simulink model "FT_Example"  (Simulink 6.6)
settings: Solver=FixedStepDiscrete  StartTime=0.0  StopTime=10  FixedStep=Ts  RelTol=1e-3
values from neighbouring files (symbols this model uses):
  Ts = 1/30    (= 0.0333333333333)    [setup.m]
libraries: RobotLibrary x2

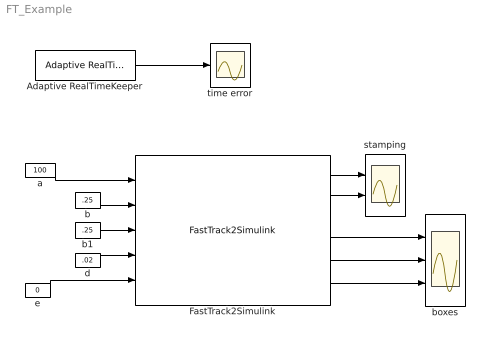
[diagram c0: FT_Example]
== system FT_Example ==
  Adaptive RealTimeKeeper : RobotLibrary/Adaptive RealTimeKeeper  Tag=AdaptiveRealTimeKeeper  Description=|  Priority=0  SystemSampleTime=-1  Ts=Ts
      | This block attempts to synchronize the simulation clock with real time.                                                                                                            
      |                                                                                                                                                                                    
      | The output provides the time-keeping err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
  FastTrack2Simulink : RobotLibrary/FastTrack2Simulink  Tag=FastTrack2Simulink  Description=Simulink interface to the FastTrack Library.  Priority=2  sampling_time=Ts  template_long_size=3  template_short_size=2  send_image_ncs=on  server_ip='128.111.56.204'  ncs_packet_id=0  rle_compress_thres=16  send_xwindows=off
  a : Constant  Value=100  SampleTime=Ts
  b : Constant  Value=.25  SampleTime=Ts
  b1 : Constant  Value=.25  SampleTime=Ts
  boxes : Scope  NumInputPorts=3
  d : Constant  Value=.02  SampleTime=Ts
  e : Constant  Value=0  SampleTime=Ts
  stamping : Scope  NumInputPorts=2
  time error : Scope
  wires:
  e/1 -> FastTrack2Simulink/5
  a/1 -> FastTrack2Simulink/1
  b/1 -> FastTrack2Simulink/2
  b1/1 -> FastTrack2Simulink/3
  d/1 -> FastTrack2Simulink/4
  Adaptive RealTimeKeeper/1 -> time error/1
  FastTrack2Simulink/1 -> stamping/1
  FastTrack2Simulink/2 -> stamping/2
  FastTrack2Simulink/3 -> boxes/1
  FastTrack2Simulink/4 -> boxes/2
  FastTrack2Simulink/5 -> boxes/3
